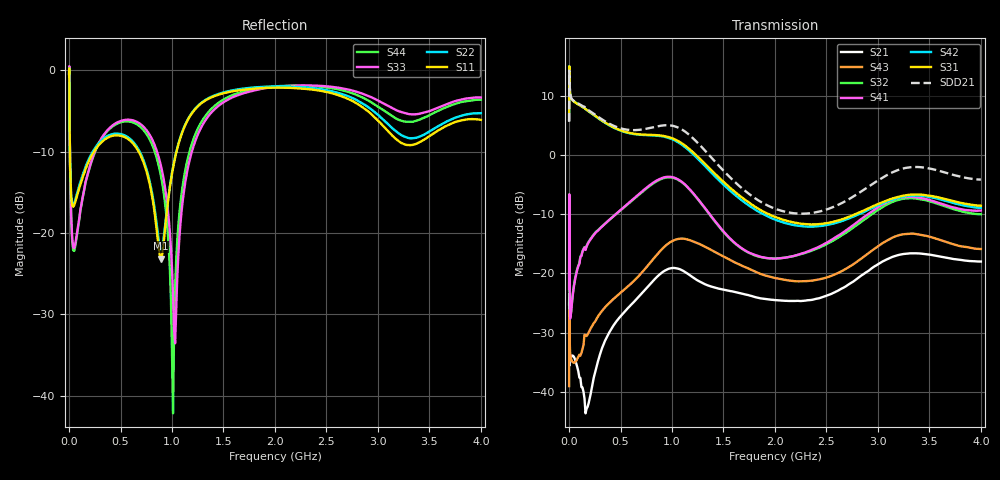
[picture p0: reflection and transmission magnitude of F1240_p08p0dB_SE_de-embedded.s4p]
! Integrated Device Technology
! Corporate Headquarters
! 6024 Silver Creek Valley Road
! San Jose, CA 95138  USA
! Phone:  1-408-284-8200
! Toll Free:  1-800-223-1366
! Webpage:  http://www.idt.com/
! Timing and RF Division
! 515 Groton Road, Suite 102
! Westford, MA 01886-6024
! Device:  F1240
! Description: Dual Intermediate Frequency Digital Variable Gain Amplifier
! Frequency:  10.0 -  500.00 MHz
! Package:  5x5 mm QFN Plastic Package: 32 pin
! Ports:  8 RF, 20 DC
!  Pin  1  = GA3 / Data  Pin 17  = RF OUT_B+
!  Pin  2  = GA4 / CLK  Pin 18  = RF OUT_B-
!  Pin  3  = GA5  Pin 19  = STBY_B
!  Pin  4  = VMODE  Pin 20  = Ground
!  Pin  5  = No Connect  Pin 21  = Ground
!  Pin  6  = GB5  Pin 22  = STB_A
!  Pin  7  = GB4  Pin 23  = RF OUT_A-  = Port 4
!  Pin  8  = GB3  Pin 24  = RF OUT_A+  = Port 3
!  Pin  9  = GB2  Pin 25  = GA0
!  Pin 10  = GB1  Pin 26  = ISET_A
!  Pin 11  = RF IN_B+  Pin 27  = VCC
!  Pin 12  = RF IN_B-  Pin 28  = Ground
!  Pin 13  = Ground  Pin 29  = RF IN_A-  = Port 2
!  Pin 14  = VCC  Pin 30  = RF IN_A+  = Port 1
!  Pin 15  = ISET_B  Pin 31  = GA1
!  Pin 16  = GB0  Pin 32  = GA2 / CSb
! Gain  = +19.5 dB
! State  = 1
! Voltage  = +5.00 V
! Current  = 85.292 mA (one channel only)
! Temperture  =  +25 C
! Test Date  =  2017-10-18
! Board  =  EB4031
! Data:  The device was measured on a custom evaluation board which has
!  individual transmission lines to the RF pins.  Data was collected
!  using a calibrated network analyzer.  The evaluation board was
!  de-embedded using Automatic Fixture Removal.
!  The reference plane is the edge of the package pin.
!  Only Channel A was measured.
!  This data is in single-ended operation.  If your needs are balanced
!  or differential S-parameters then this file needs to be used a
!  linear simulator.
! File Date:  2017-11-10  MJV
! Note:
!  Integrated Device Technology supplies this data as a sample of measured
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# Hz S dB R 100
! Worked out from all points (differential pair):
!   410 points, 500 kHz to 4 GHz, reference 100 ohm
!   strongest paths, dB at 500 kHz, 930 MHz, 1.96 GHz, 2.98 GHz, 4 GHz:
!     S31: 5.9, 3.2, -10.2, -8.5, -8.6
!     S42: 5.9, 3.0, -10.6, -8.7, -9.0
!     S41: -22.6, -3.8, -17.5, -9.1, -9.4
!     S32: -22.9, -3.9, -17.5, -9.5, -10.0
!     S43: -39.1, -15.5, -20.6, -15.7, -15.9
!     S21: -25.2, -19.6, -24.5, -18.7, -18.0
!   taken as a pair (ports 1,2 in; 3,4 out), SDD21 dB: 5.6, 5.0, -8.8, -4.6, -4.2
!   lowest |S11| = -23.2 dB at 890 MHz (marker M1), VSWR 1.15, Z = 111 + j9.74 ohm
!   |S11| at or under -10 dB: 8.434 MHz to 243.3 MHz (234.8 MHz wide, 187 % of centre); 675.4 MHz to 1.043 GHz (368 MHz wide, 42.8 % of centre)
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500000  -0.42 -5.6  -25.25 -5.3  -27.18 82.5  -57.81 70.4
        -25.25 -5.4  -0.42 -5.5  -57.97 68.2  -27.17 83.6
        5.89 -105.1  -22.88 -86.9  -0.50 1.4  -39.13 -93.3
        -22.60 -86.7  5.87 -103.9  -39.06 -93.4  -0.51 3.8
3000000  -2.60 -59.5  -31.20 -79.9  -15.59 26.6  -53.25 -52.0
         -31.27 -79.0  -2.56 -59.5  -53.23 -52.5  -15.60 26.8
         14.19 179.6  -11.50 149.1  -2.07 -54.9  -27.17 -175.1
         -11.64 148.8  14.18 179.8  -27.14 -175.0  -2.13 -54.7
3e7  -16.64 -109.6  -33.80 -10.1  -15.83 -7.9  -48.34 64.2
     -33.88 -10.4  -16.44 -109.9  -48.16 64.7  -15.81 -7.8
     9.28 163.1  -24.50 58.8  -20.64 -91.4  -35.17 160.2
     -24.66 58.0  9.31 163.1  -34.90 160.2  -20.96 -91.0
2e8  -10.99 -139.2  -41.89 20.7  -17.39 -50.2  -34.16 23.6
     -41.16 22.7  -10.73 -140.0  -34.15 24.4  -17.41 -50.3
     7.25 109.8  -14.40 7.4  -11.90 -103.8  -30.02 104.4
     -14.50 7.1  7.23 109.1  -29.67 103.0  -11.97 -102.8
8.9e8  -23.16 38.9  -20.28 -86.2  -16.46 171.8  -25.79 -139.5
       -20.05 -91.4  -22.11 40.0  -26.01 -132.7  -16.72 171.2
       3.26 -63.9  -4.13 -172.7  -11.63 136.0  -16.90 -68.8
       -4.00 -176.3  3.16 -65.6  -16.15 -71.3  -12.84 136.5
1.21e9  -5.02 -113.3  -20.09 -176.6  -18.68 83.4  -25.30 145.4
        -20.77 179.6  -4.96 -112.9  -24.87 152.4  -19.29 82.3
        0.34 -158.3  -6.63 74.3  -9.29 -99.2  -15.14 -167.9
        -6.57 69.5  0.02 -160.1  -14.64 -170.4  -8.43 -103.7
4e9  -6.11 -150.5  -18.13 83.3  -20.37 -66.2  -21.27 -48.0
     -18.02 82.6  -5.29 -147.8  -22.43 -28.4  -22.08 -58.9
     -8.60 23.8  -10.04 -93.0  -3.36 -139.6  -16.99 83.0
     -9.40 -107.3  -8.96 31.5  -15.90 59.2  -3.62 -147.1
